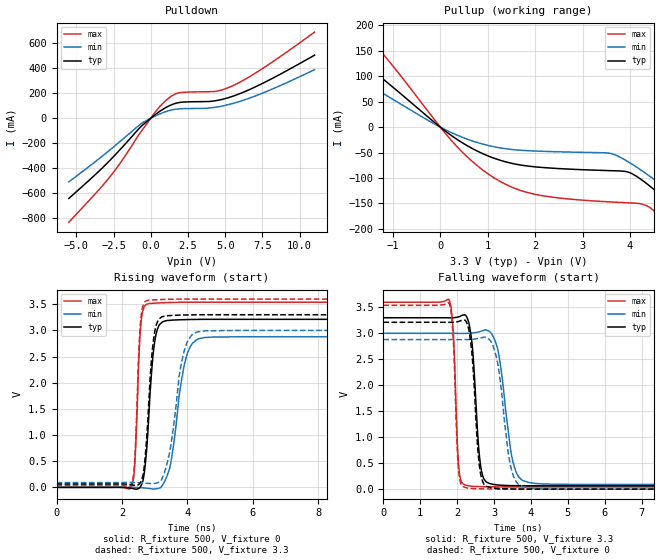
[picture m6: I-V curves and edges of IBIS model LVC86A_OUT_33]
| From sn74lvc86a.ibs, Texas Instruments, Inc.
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[Model]   LVC86A_OUT_33
Model_type  Output
Vref =   0
Rref =   500
Cref =   50p
Vmeas =   1.5
| variable   typ   min   max
C_comp   5.73pF   3.46pF   7.15pF
| C_pullup   5.72pF   3.46pF   7.15pF
| C_pulldown   5.74pF   4.21pF   7.10pF
[Temperature Range]   40   100   -40
| Ambient temperature   25   85   -40
[Voltage range]   3.3   3   3.6
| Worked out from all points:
|   slope of the pulldown table from 0 to 0.495 V, typ, clamps not added: 10.7 ohm
|   slope of the pullup table from 0 to 0.495 V, typ, clamps not added: 15.2 ohm
|   rising waveform, R_fixture 500, V_fixture 0: 20-80 % time 213ps typ, 373ps min, 132ps max; typ from 0 V to 3.21 V
|   falling waveform, R_fixture 500, V_fixture 3.3: 20-80 % time 171ps typ, 302ps min, 109ps max; typ from 3.3 V to 0.065 V
|   rising waveform, R_fixture 500, V_fixture 3.3: 20-80 % time 206ps typ, 376ps min, 129ps max; typ from 0.065 V to 3.3 V
|   falling waveform, R_fixture 500, V_fixture 0: 20-80 % time 169ps typ, 286ps min, 108ps max; typ from 3.21 V to 0 V
[Pulldown]
| LVC86A_OUT_33
|   Voltage   I(typ)   I(min)   I(max)
-5.5V     -642.1mA   -509.2mA   -832.1mA
-3.645V   -442.6mA   -340.3mA   -594.1mA
-2.71V    -333.2mA   -250.5mA   -464.6mA
-1.885V   -228.4mA   -168.1mA   -330.7mA
-620mV    -62.4mA    -41.49mA   -102.1mA
455mV     42.83mA    26.93mA    71.74mA
1.215V    98.07mA    60.46mA    162.3mA
1.91V     125.9mA    75.23mA    203.5mA
4.31V     139.6mA    87.57mA    214.6mA
5.45V     173.8mA    116.3mA    257.3mA
7.53V     280.4mA    202.4mA    399.9mA
11V       505.3mA    389mA      689.8mA
[Pullup]
| LVC86A_OUT_33
|   Voltage   I(typ)   I(min)   I(max)
-5.5V     404.4mA    310.8mA    569.2mA
-3.515V   265mA      197.3mA    383.4mA
-2.48V    190.1mA    138.3mA    280.1mA
-1.635V   127.1mA    90.28mA    191.1mA
505mV     -33.05mA   -21.44mA   -52.79mA
1.855V    -76.61mA   -46.34mA   -128.9mA
3.7V      -85.85mA   -55.1mA    -147.6mA
4.24V     -103.3mA   -84.95mA   -151mA
4.895V    -154.7mA   -130.6mA   -201.2mA
5.365V    -197.4mA   -166.8mA   -253mA
5.825V    -241.6mA   -203.9mA   -307.6mA
11V       -786.6mA   -661.2mA   -974mA
[Ramp]
| LVC86A_OUT_33
| variable   typ   min   max
dV/dt_r   1.95/2.25E-10   1.75/3.93E-10   2.14/1.39E-10
dV/dt_f   1.97/1.80E-10   1.79/3.33E-10   2.17/1.13E-10
R_load = 500
[Rising Waveform]
| LVC86A_OUT_33
R_fixture =   500
C_fixture =   0
L_fixture =   0
V_fixture =   0
V_fixture_min = 0
V_fixture_max = 0
|   Time   V(typ)   V(min)   V(max)
0s        184.9pV    3.596nV    20.95pV
2.29ns    -17.24mV   1.254mV    10.63mV
2.395ns   -30.28mV   299.2uV    456.8mV
2.58ns    25.66mV    -6.539mV   3.117V
2.82ns    1.328V     -20.22mV   3.512V
3.13ns    3.09V      -15.76mV   3.526V
3.47ns    3.194V     385.2mV    3.535V
3.96ns    3.207V     2.471V     3.539V
4.375ns   3.212V     2.846V     3.539V
24.99ns   3.212V     2.88V      3.539V
[Falling Waveform]
| LVC86A_OUT_33
R_fixture =   500
C_fixture =   0
L_fixture =   0
V_fixture =   3.3
V_fixture_min = 3
V_fixture_max = 3.6
|   Time   V(typ)   V(min)   V(max)
0s        3.3V       3V         3.6V
1.785ns   3.299V     3V         3.638V
1.9ns     3.301V     3V         2.967V
2.055ns   3.321V     2.999V     348.7mV
2.28ns    3.281V     3V         66.4mV
2.64ns    429.4mV    3.039V     47.93mV
2.975ns   91.17mV    2.941V     44.04mV
3.515ns   66.56mV    516.4mV    42.1mV
3.945ns   64.24mV    126.1mV    41.88mV
24.99ns   64.52mV    92.1mV     41.93mV
[Rising Waveform]
| LVC86A_OUT_33
R_fixture =   500
C_fixture =   0
L_fixture =   0
V_fixture =   3.3
V_fixture_min = 3
V_fixture_max = 3.6
|   Time   V(typ)   V(min)   V(max)
0s        64.52mV    92.1mV     41.93mV
2.29ns    48.66mV    93.04mV    60.34mV
2.39ns    39mV       92.1mV     494.2mV
2.57ns    97.74mV    86.04mV    3.167V
2.765ns   1.02V      77.93mV    3.572V
3.07ns    3.138V     84.25mV    3.587V
3.46ns    3.284V     671.1mV    3.596V
3.91ns    3.295V     2.617V     3.599V
4.34ns    3.3V       2.977V     3.6V
24.99ns   3.3V       3V         3.6V
[Falling Waveform]
| LVC86A_OUT_33
R_fixture =   500
C_fixture =   0
L_fixture =   0
V_fixture =   0
V_fixture_min = 0
V_fixture_max = 0
|   Time   V(typ)   V(min)   V(max)
0s        3.212V     2.88V      3.539V
1.78ns    3.212V     2.879V     3.577V
1.9ns     3.214V     2.879V     2.815V
2.04ns    3.229V     2.879V     351.7mV
2.28ns    3.165V     2.88V      20.41mV
2.61ns    410.4mV    2.906V     5.948mV
2.905ns   30.28mV    2.853V     2.411mV
3.46ns    2.243mV    407.8mV    250.2uV
3.855ns   96.19uV    29.84mV    -8.173uV
24.99ns   4.215nV    20.62nV    4.114nV
